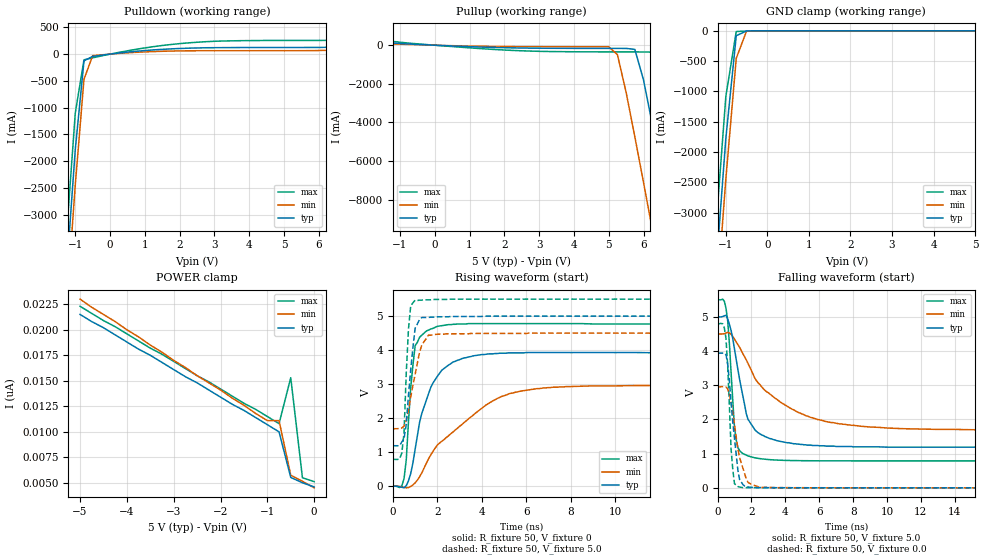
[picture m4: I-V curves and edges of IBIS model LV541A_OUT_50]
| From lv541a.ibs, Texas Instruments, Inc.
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|   Model LV541A_OUT_50
[Model]   LV541A_OUT_50
Model_type  3-state
Polarity   Non-Inverting
Enable   Active-Low
Vinl = 1.5
Vinh = 3.5
Vmeas = 2.5v
Cref = 15pf
| variable   typ   min   max
C_comp   4.60pf   3.45pf   5.75pf
[Temperature Range]   25   85   -40
[Voltage Range]   5.0   4.5   5.5
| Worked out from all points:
|   slope of the pulldown table from 0 to 0.75 V, typ, clamps not added: 14.1 ohm
|   slope of the pullup table from 0 to 0.75 V, typ, clamps not added: 13 ohm
|   GND clamp passes 1 mA (typ) near -0.47 V on its own axis
|   rising waveform, R_fixture 50, V_fixture 0: 20-80 % time 981ps typ, 2.7ns min, 329ps max; typ from 0 V to 3.92 V
|   falling waveform, R_fixture 50, V_fixture 5.0: 20-80 % time 928ps typ, 3.11ns min, 360ps max; typ from 5 V to 1.19 V
|   rising waveform, R_fixture 50, V_fixture 5.0: 20-80 % time 314ps typ, 494ps min, 187ps max; typ from 1.19 V to 5 V
|   falling waveform, R_fixture 50, V_fixture 0.0: 20-80 % time 448ps typ, 643ps min, 264ps max; typ from 3.94 V to 0 V
[Pulldown]
|   Voltage   I(typ)   I(min)   I(max)
-5V       -41A       -41.6A     -40.3A
-1.25V    -4.06A     -4.73A     -3.36A
-1V       -1.78A     -2.44A     -1.1A
-750mV    -126mA     -470mA     -106mA
-500mV    -41.9mA    -28.2mA    -69.2mA
1V        67mA       41.6mA     116mA
2.25V     111mA      62mA       210mA
3.25V     121mA      63.6mA     245mA
6.75V     138mA      78.4mA     266mA
8V        176mA      104mA      321mA
10V       253mA      150mA      452mA
[Pullup]
|   Voltage   I(typ)   I(min)   I(max)
-5V       414mA      225mA      775mA
1.5V      -105mA     -57.9mA    -197mA
5V        -164mA     -78.5mA    -346mA
5.25V     -164mA     -487mA     -346mA
5.75V     -214mA     -4.74A     -346mA
6V        -1.8A      -7.11A     -349mA
6.25V     -4.07A     -9.52A     -356mA
6.5V      -6.45A     -11.9A     -1.14A
6.75V     -8.86A     -14.4A     -3.37A
7.25V     -13.8A     -19.3A     -8.18A
7.5V      -16.2A     -21.8A     -10.6A
10V       -41A       -46.5A     -35.4A
[GND Clamp]
|   Voltage   I(typ)   I(min)   I(max)
-5V       -41A       -41.6A     -40.3A
-1.25V    -4.06A     -4.73A     -3.35A
-1V       -1.77A     -2.44A     -1.08A
-750mV    -80.8mA    -454mA     -11.4mA
-500mV    -1.16mA    -866uA     -3.99mA
5V        4.6nA      5.75nA     4.37nA
[POWER Clamp]
|   Voltage   I(typ)   I(min)   I(max)
-5V       21.5nA     23nA       22.3nA
-3.5V     17.5nA     18.5nA     18.2nA
-2.75V    15.4nA     16.3nA     16.2nA
-2.5V     14.8nA     15.5nA     15.5nA
-1.75V    12.7nA     13.3nA     13.5nA
-1.5V     12.1nA     12.6nA     12.8nA
-1.25V    11.4nA     11.8nA     12.2nA
-1V       10.7nA     11.1nA     11.5nA
-750mV    10nA       11.1nA     10.8nA
-500mV    5.53nA     5.75nA     15.3nA
-250mV    5.01nA     5.16nA     5.5nA
0V        4.6nA      4.51nA     5.12nA
[Ramp]
| variable   typ   min   max
dV/dt_r   2.36E+00/9.94E-10   1.78E+00/2.72E-09   2.86E+00/3.11E-10
dV/dt_f   2.32E+00/9.23E-10   1.72E+00/3.09E-09   2.56E+00/4.42E-10
R_load = 50
[Rising Waveform]
R_fixture = 50
V_fixture = 0
|   Time   V(typ)   V(min)   V(max)
0s        0V         0V         0V
500ps     -44.8mV    -36mV      226mV
600ps     15.5mV     -48.4mV    775mV
800ps     373mV      -8.92mV    2.89V
1ns       1.09V      99.2mV     4.13V
1.3ns     2.14V      394mV      4.44V
2ns       3.23V      1.21V      4.7V
4.5ns     3.89V      2.51V      4.78V
6.5ns     3.93V      2.87V      4.78V
25ns      3.92V      2.95V      4.77V
[Falling Waveform]
R_fixture = 50
V_fixture = 5.0
V_fixture_min = 4.5
V_fixture_max = 5.5
|   Time   V(typ)   V(min)   V(max)
0s        5V         4.5V       5.5V
400ps     5.03V      4.51V      5.46V
600ps     4.94V      4.55V      4.88V
1ns       4.06V      4.35V      1.76V
1.1ns     3.76V      4.27V      1.4V
1.8ns     2V         3.64V      935mV
2.4ns     1.61V      3.07V      863mV
3.7ns     1.36V      2.51V      809mV
6.7ns     1.22V      1.91V      790mV
25ns      1.19V      1.69V      788mV
[Rising Waveform]
R_fixture = 50
V_fixture = 5.0
V_fixture_min = 4.5
V_fixture_max = 5.5
|   Time   V(typ)   V(min)   V(max)
0s        1.19V      1.69V      788mV
400ps     1.3V       1.71V      976mV
500ps     1.4V       1.77V      1.58V
600ps     1.82V      1.94V      3.33V
700ps     2.68V      2.23V      4.62V
800ps     3.42V      2.61V      5.3V
1ns       4.65V      3.29V      5.47V
1.3ns     4.96V      4.15V      5.47V
2ns       4.98V      4.47V      5.49V
25ns      5V         4.5V       5.5V
[Falling Waveform]
R_fixture = 50
V_fixture = 0.0
|   Time   V(typ)   V(min)   V(max)
0s        3.94V      2.95V      4.8V
300ps     3.94V      2.96V      4.8V
500ps     3.89V      2.95V      4.36V
600ps     3.62V      2.89V      3.54V
800ps     2.47V      2.49V      1.12V
1ns       1.44V      1.85V      118mV
1.2ns     516mV      1.14V      40.5mV
1.8ns     25.5mV     161mV      7.82mV
2.5ns     8.07mV     15.1mV     3.06mV
25ns      50.9uV     54.9uV     57.6uV
